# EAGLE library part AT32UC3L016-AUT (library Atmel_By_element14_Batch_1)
MCU
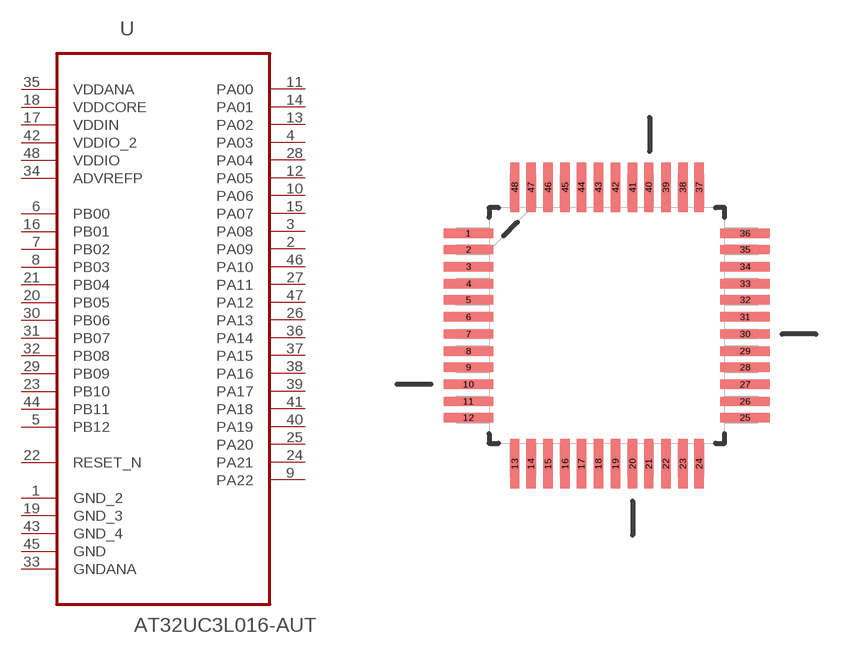
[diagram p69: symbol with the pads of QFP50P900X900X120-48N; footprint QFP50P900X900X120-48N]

Designator prefix U

## AT32UC3L016-AUT (DESCRIPTION: MCU; MPN: AT32UC3L016-AUT; OC_FARNELL: 1841643; OC_NEWARK: 12T1378; PACKAGE: QFP-48; SUPPLIER: Atmel)  [QFP50P900X900X120-48N]
1  GND_2  pas
2  PA09
3  PA08
4  PA03
5  PB12
6  PB00
7  PB02
8  PB03
9  PA22
10  PA06
11  PA00
12  PA05
13  PA02
14  PA01
15  PA07
16  PB01
17  VDDIN  pwr
18  VDDCORE  pwr
19  GND_3  pas
20  PB05
21  PB04
22  RESET_N  in
23  PB10
24  PA21
25  PA20
26  PA13
27  PA11
28  PA04
29  PB09
30  PB06
31  PB07
32  PB08
33  GNDANA  pas
34  ADVREFP  pwr
35  VDDANA  pwr
36  PA14
37  PA15
38  PA16
39  PA17
40  PA19
41  PA18
42  VDDIO_2  pwr
43  GND_4  pas
44  PB11
45  GND  pas
46  PA10
47  PA12
48  VDDIO  pwr

## Footprint QFP50P900X900X120-48N (pad centres in mm)
smd 1.473 x 0.279: 1 -4.115,2.743; 2 -4.115,2.261; 3 -4.115,1.753; 4 -4.115,1.245; 5 -4.115,0.762; 6 -4.115,0.254; 7 -4.115,-0.254; 8 -4.115,-0.762; 9 -4.115,-1.245; 10 -4.115,-1.753; 11 -4.115,-2.261; 12 -4.115,-2.743; 25 4.115,-2.743; 26 4.115,-2.261; 27 4.115,-1.753; 28 4.115,-1.245; 29 4.115,-0.762; 30 4.115,-0.254; 31 4.115,0.254; 32 4.115,0.762; 33 4.115,1.245; 34 4.115,1.753; 35 4.115,2.261; 36 4.115,2.743
smd 0.279 x 1.473: 13 -2.743,-4.115; 14 -2.261,-4.115; 15 -1.753,-4.115; 16 -1.245,-4.115; 17 -0.762,-4.115; 18 -0.254,-4.115; 19 0.254,-4.115; 20 0.762,-4.115; 21 1.245,-4.115; 22 1.753,-4.115; 23 2.261,-4.115; 24 2.743,-4.115; 37 2.743,4.115; 38 2.261,4.115; 39 1.753,4.115; 40 1.245,4.115; 41 0.762,4.115; 42 0.254,4.115; 43 -0.254,4.115; 44 -0.762,4.115; 45 -1.245,4.115; 46 -1.753,4.115; 47 -2.261,4.115; 48 -2.743,4.115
